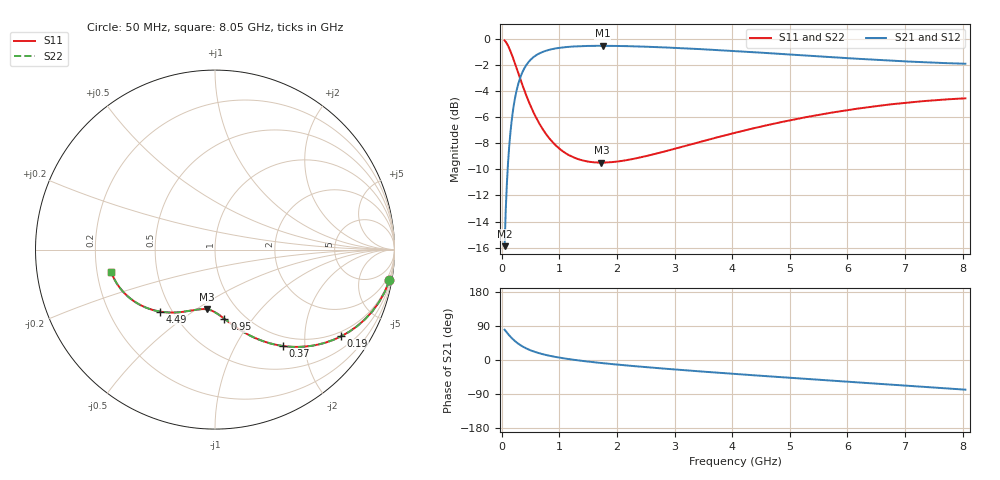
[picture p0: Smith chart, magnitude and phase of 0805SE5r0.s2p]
! AVX Thin Film Operation		Date: August 2001
! Description: Accu-P® Series, Thin Film, SMD, RF Capacitor
! Part Number: 08051J5R0ABT
! 50 MHz  -  8.05 GHz
! Serial Measurements
# mhz S db R 50
!	S11		S21		S12		S22
!	dB	Phase	dB	Phase	dB	Phase	dB	Phase
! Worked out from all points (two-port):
!   401 points, 50 MHz to 8.05 GHz, reference 50 ohm
!   highest |S21| = -0.52 dB at 1.75 GHz (marker M1); lowest = -15.9 dB at 50 MHz (marker M2)
!   |S21| within 3 dB of the highest: 282.5 MHz to end of sweep
!   lowest |S11| = -9.5 dB at 1.73 GHz (marker M3), VSWR 2.01, Z = 36.8 - j27.6 ohm
!   |S11| at or under -10 dB: nowhere
!   |S22| runs from -9.5 to -0.1 dB; largest |S21 - S12| = 0
!   S11 on the Smith chart (normalised r, x): 50 MHz: 1, -11; 190 MHz: 0.85, -3.01; 370 MHz: 0.84, -1.59; 950 MHz: 0.81, -0.74; 4.49 GHz: 0.43, -0.38; 8.05 GHz: 0.26, -0.10
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50  -0.11 -10.0  -15.89 80.0  -15.89 80.0  -0.11 -10.0
90  -0.36 -17.7  -11.04 72.3  -11.04 72.3  -0.36 -17.7
110  -0.52 -21.4  -9.48 68.6  -9.48 68.6  -0.52 -21.4
130  -0.71 -24.9  -8.23 65.1  -8.23 65.1  -0.71 -24.9
190  -1.38 -34.5  -5.66 55.5  -5.66 55.5  -1.38 -34.5
270  -2.40 -44.9  -3.73 45.0  -3.73 45.0  -2.40 -45.0
370  -3.67 -54.9  -2.44 35.0  -2.44 35.0  -3.67 -55.0
490  -5.02 -63.7  -1.64 26.3  -1.64 26.3  -5.02 -63.7
610  -6.14 -70.2  -1.21 19.8  -1.21 19.8  -6.14 -70.2
770  -7.29 -76.7  -0.90 13.2  -0.90 13.2  -7.29 -76.7
950  -8.21 -82.3  -0.71 7.6  -0.71 7.6  -8.21 -82.3
1390  -9.30 -92.1  -0.55 -2.2  -0.55 -2.2  -9.30 -92.1
1730  -9.48 -97.9  -0.52 -8.0  -0.52 -8.0  -9.48 -97.9
1750  -9.48 -98.2  -0.52 -8.3  -0.52 -8.3  -9.48 -98.2
2210  -9.26 -104.9  -0.55 -15.0  -0.55 -15.0  -9.26 -104.9
2730  -8.74 -111.5  -0.63 -21.6  -0.63 -21.6  -8.74 -111.6
3370  -7.98 -119.1  -0.76 -29.2  -0.76 -29.2  -7.98 -119.1
4050  -7.20 -126.7  -0.93 -36.8  -0.93 -36.8  -7.20 -126.7
4490  -6.73 -131.4  -1.05 -41.5  -1.05 -41.5  -6.73 -131.4
5390  -5.91 -140.8  -1.30 -51.0  -1.30 -51.0  -5.91 -140.8
6730  -5.03 -154.5  -1.66 -64.7  -1.66 -64.7  -5.03 -154.5
8050  -4.55 -168.1  -1.90 -78.3  -1.90 -78.3  -4.55 -168.1
